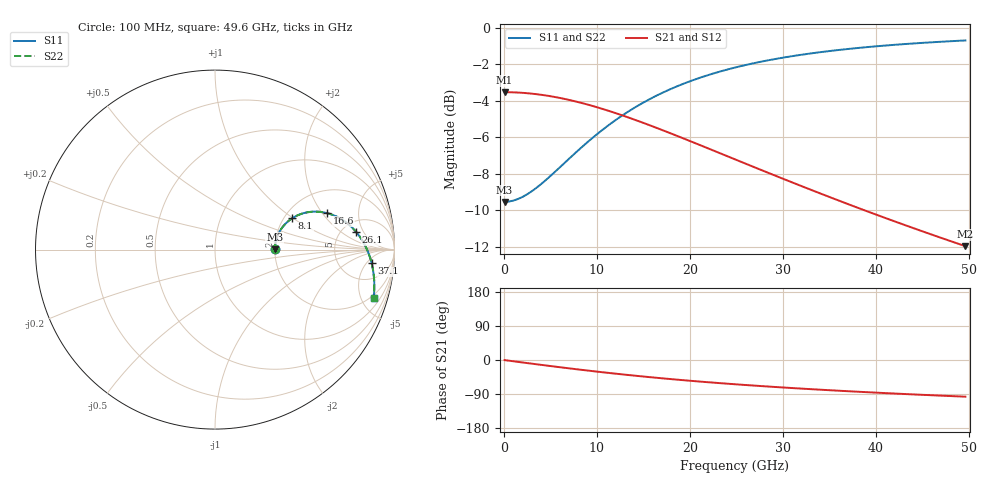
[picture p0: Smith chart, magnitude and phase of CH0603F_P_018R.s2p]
# GHz S RI R 18
! S-Parameters data
! Freq  reS11  imS11  reS21  imS21  reS12  imS12  reS22  imS22
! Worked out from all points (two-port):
!   100 points, 100 MHz to 49.6 GHz, reference 18 ohm
!   highest |S21| = -3.52 dB at 100 MHz (marker M1); lowest = -12.0 dB at 49.6 GHz (marker M2)
!   |S21| within 3 dB of the highest: start of sweep to 21.56 GHz
!   lowest |S11| = -9.5 dB at 100 MHz (marker M3), VSWR 2.00, Z = 36 + j0.211 ohm
!   |S11| at or under -10 dB: nowhere
!   |S22| runs from -9.5 to -0.7 dB; largest |S21 - S12| = 0
!   S11 on the Smith chart (normalised r, x): 100 MHz: 2.00, +0.01; 8.1 GHz: 2.21, +0.98; 16.6 GHz: 3.11, +2.22; 26.1 GHz: 6.72, +3.56; 37.1 GHz: 11, -7; 49.6 GHz: 1.69, -6.26
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0.1  0.3334 0.00261  0.6666 -0.00374  0.6666 -0.00374  0.3334 0.00261
1.6  0.3376 0.0414  0.6622 -0.0595  0.6622 -0.0595  0.3376 0.0414
3.1  0.3491 0.0785  0.6503 -0.1136  0.6503 -0.1136  0.3491 0.0785
4.1  0.3605 0.1017  0.6384 -0.148  0.6384 -0.148  0.3605 0.1017
5.6  0.3826 0.1331  0.6154 -0.1964  0.6154 -0.1964  0.3826 0.1331
8.1  0.4299 0.1745  0.5659 -0.2659  0.5659 -0.2659  0.4299 0.1745
8.6  0.4405 0.181  0.5548 -0.278  0.5548 -0.278  0.4405 0.181
10.6  0.4854 0.2006  0.5075 -0.32  0.5075 -0.32  0.4854 0.2006
12.6  0.5322 0.2103  0.4577 -0.352  0.4577 -0.352  0.5322 0.2103
14.6  0.5787 0.2109  0.4078 -0.3749  0.4078 -0.3749  0.5787 0.2109
16.6  0.6233 0.2035  0.3593 -0.3896  0.3593 -0.3896  0.6233 0.2035
18.6  0.6649 0.1895  0.3133 -0.3976  0.3133 -0.3976  0.6649 0.1895
20.6  0.7028 0.1702  0.2705 -0.4001  0.2705 -0.4001  0.7028 0.1702
22.6  0.7367 0.1467  0.2312 -0.3982  0.2312 -0.3982  0.7367 0.1467
25.1  0.7734 0.1129  0.1871 -0.3912  0.1871 -0.3912  0.7734 0.1129
26.1  0.7863 0.0984  0.171 -0.3873  0.171 -0.3873  0.7863 0.0984
29.6  0.8244 0.0447  0.1211 -0.3703  0.1211 -0.3703  0.8244 0.0447
33.1  0.852 -0.0116  0.0803 -0.3501  0.0803 -0.3501  0.852 -0.0116
37.1  0.8729 -0.0766  0.0428 -0.3253  0.0428 -0.3253  0.8729 -0.0766
41.6  0.885 -0.1486  0.0101 -0.2972  0.0101 -0.2972  0.885 -0.1486
45.6  0.8875 -0.2104  -0.0122 -0.2732  -0.0122 -0.2732  0.8875 -0.2104
49.6  0.8838 -0.2697  -0.0297 -0.2504  -0.0297 -0.2504  0.8838 -0.2697
